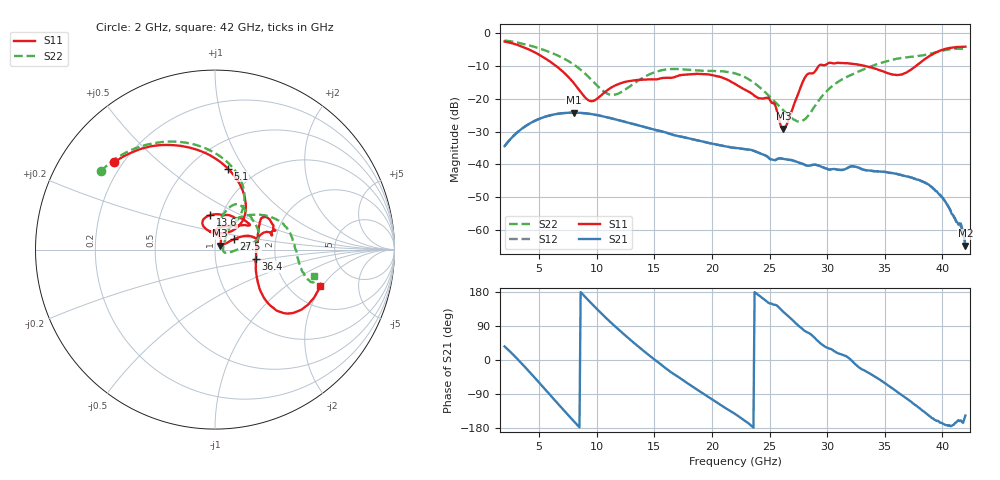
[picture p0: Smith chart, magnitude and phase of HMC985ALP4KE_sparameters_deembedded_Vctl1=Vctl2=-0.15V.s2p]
!s2p File: Measurements: S11, S21, S12, S22
# GHz S dB R 50.0
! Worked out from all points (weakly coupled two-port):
!   401 points, 2 GHz to 42 GHz, reference 50 ohm
!   highest |S21| = -24.22 dB at 8 GHz (marker M1); lowest = -64.7 dB at 42 GHz (marker M2)
!   lowest |S11| = -29.1 dB at 26.2 GHz (marker M3), VSWR 1.07, Z = 52.8 + j2.31 ohm
!   |S11| at or under -10 dB: 6.46 GHz to 29.27 GHz (22.81 GHz wide, 128 % of centre); 33.28 GHz to 37.72 GHz (4.443 GHz wide, 12.5 % of centre)
!   |S22| runs from -26.9 to -2.2 dB; largest |S21 - S12| = 0.00013
!   S11 on the Smith chart (normalised r, x): 2 GHz: 0.17, +0.36; 5.1 GHz: 0.74, +0.85; 13.6 GHz: 0.88, +0.35; 27.5 GHz: 1.23, +0.14; 36.4 GHz: 1.58, -0.17; 42 GHz: 2.91, -1.91
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2  -2.58 139.2  -34.40 35.7  -34.42 35.8  -2.25 145.6
3.5  -4.11 111.1  -29.10 -9.9  -29.11 -9.8  -3.20 121.9
5.1  -6.81 80.9  -25.98 -63.2  -25.98 -63.2  -4.76 97.5
8  -15.20 45.1  -24.22 -161.3  -24.22 -161.3  -9.56 60.4
8.7  -18.39 52.9  -24.32 175.9  -24.33 175.8  -11.45 55.2
9.6  -20.72 85.8  -24.69 147.3  -24.70 147.3  -14.42 52.9
11.2  -16.72 116.3  -25.89 99.6  -25.90 99.6  -18.75 68.2
13.6  -14.26 98.2  -28.08 35.7  -28.09 35.7  -14.46 77.8
15.4  -13.93 73.2  -29.72 -7.6  -29.73 -7.6  -11.51 68.3
19.4  -12.52 35.2  -33.18 -91.9  -33.18 -91.9  -11.50 34.4
22  -15.45 52.7  -34.95 -142.3  -34.96 -142.3  -12.28 13.5
25  -20.16 96.2  -38.21 149.6  -38.22 149.5  -19.31 -3.4
26.2  -29.11 38.5  -38.30 127.1  -38.30 127.1  -23.53 -15.5
27.5  -18.31 28.3  -39.34 90.8  -39.34 90.6  -26.87 -3.1
28.1  -13.35 20.1  -40.17 75.9  -40.17 75.9  -26.13 20.0
28.7  -12.27 12.3  -40.12 64.8  -40.16 65.3  -23.44 38.3
31  -9.08 22.9  -41.62 17.1  -41.60 17.1  -14.71 56.4
35.4  -12.35 12.2  -42.52 -69.3  -42.55 -69.6  -8.37 26.0
36.4  -12.66 -12.9  -43.14 -90.9  -43.18 -91.1  -7.60 17.3
39.7  -5.49 -42.0  -49.02 -162.4  -48.82 -163.3  -5.63 -16.5
41.5  -4.20 -23.0  -57.90 -161.3  -58.21 -163.5  -4.74 -17.7
42  -4.15 -18.9  -64.75 -146.5  -64.86 -152.1  -4.89 -14.8
